(* Logix 5000 AddOnInstructionDefinition export AMCI_MA_Run_Dwell_Move; software revision 20.05 *)

TYPE AMCI_Motion_Axis_Output_Data :
STRUCT
   Control_Word_0 : INT;
   Control_Word_1 : INT;
   Position_or_Distance : DINT;
   Programmed_Speed : DINT;
   Acceleration : INT;
   Deceleration : INT;
   Output_Word_8 : INT;
   Output_Word_9 : INT;
END_STRUCT
END_TYPE

TYPE AMCI_Motion_Axis_Input_Data :
STRUCT
   Moving_CW : BOOL;
   Moving_CCW : BOOL;
   In_Hold_State : BOOL;
   Stopped : BOOL;
   At_Home : BOOL;
   Accelerating : BOOL;
   Decelerating : BOOL;
   Move_Complete : BOOL;
   Status_Word_0_Bit_8 : BOOL;
   Status_Word_0_Bit_9 : BOOL;
   Position_Invalid : BOOL;
   Input_Error : BOOL;
   Command_Error : BOOL;
   Configuration_Error : BOOL;
   Module_OK : BOOL;
   Mode_Flag : BOOL;
   IN1_Active : BOOL;
   IN2_Active : BOOL;
   IN3_Active : BOOL;
   IN4_Active : BOOL;
   Status_Word_1_Bit_4 : BOOL;
   Status_Word_1_Bit_5 : BOOL;
   Connection_Was_Lost : BOOL;
   Driver_Fault : BOOL;
   Status_Word_1_Bit_8 : BOOL;
   Invalid_Jog_Change : BOOL;
   Status_Word_1_Bit_10 : BOOL;
   Heartbeat_Bit : BOOL;
   Status_Word_1_Bit_12 : BOOL;
   Status_Word_1_Bit_13 : BOOL;
   Stall_Detected : BOOL;
   Drive_Is_Enabled : BOOL;
   Motor_Position : DINT;
   Encoder_Position : DINT;
   Trapped_Encoder_Position : DINT;
   Input_Word_8 : INT;
   Input_Word_9 : INT;
END_STRUCT
END_TYPE

ADD_ON_INSTRUCTION AMCI_MA_Run_Dwell_Move   (* revision 1.0, vendor AMCI, ExecuteEnableInFalse *)
// Run Dwell Moves for SD and SMD devices.  Will not work with SV integrated servo devices.
// Help:
// MOTION AXIS RUN DWELL MOVE
// This AOI will only work with the SD and SMD motion devices.  The SV motion devices do not support Assembled Moves.
// AXIS INPUT DATA:  Input data from AMCI motion device.   Uses the AMCI_Motion_Axis_Input_Data User Defined Data Type.
// AXIS OUTPUT DATA; Output data from the AOI to the AMCI motion device.   Uses the AMCI_Motion_Axis_Output_Data User Defined Data Type.
// DWELL TIME:Time in milliseconds between each of the assembled move segments.
// EN (Enable) Set when rung is true, Reset when rung is false
// DN (Done) Set when command is sent to the motion device.  Reset when the rung is false.
// ER (Error) Set when a command or input error failed to clear.  Reset when the rung is false.
// IP (In Process) Set when motion is occurring.   Reset when motion stops or the rung goes false.
VAR_IN_OUT
   Axis_Input_Data : AMCI_Motion_Axis_Input_Data; {required}
   Axis_Output_Data : AMCI_Motion_Axis_Output_Data; {required}
END_VAR
VAR_INPUT
   Type_0_for_standard_1_for_indexed : BOOL;
   Dwell_Time : INT; {required}
END_VAR
VAR_OUTPUT
   EN : BOOL; {visible}
   DN : BOOL; {visible}
   ER : BOOL; {visible}
   IP : BOOL; {visible}
END_VAR
VAR
   command_data_block : INT[10];
        [0]   // Command Bits MSW
        [1]   // Command Bits LSW
        [2]   // Upper Target Position
        [3]   // Lower Target Position
        [4]   // Upper Programmed Speed
        [5]   // Lower Programmed Speed
END_VAR

ROUTINE EnableInFalse   (* ladder *)
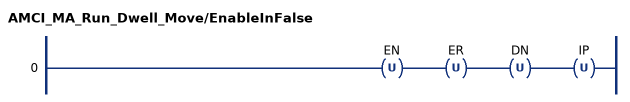
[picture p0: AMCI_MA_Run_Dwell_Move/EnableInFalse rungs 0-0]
   0: OTU(EN)OTU(ER)OTU(DN)OTU(IP);
END_ROUTINE

ROUTINE Logic   (* ladder *)
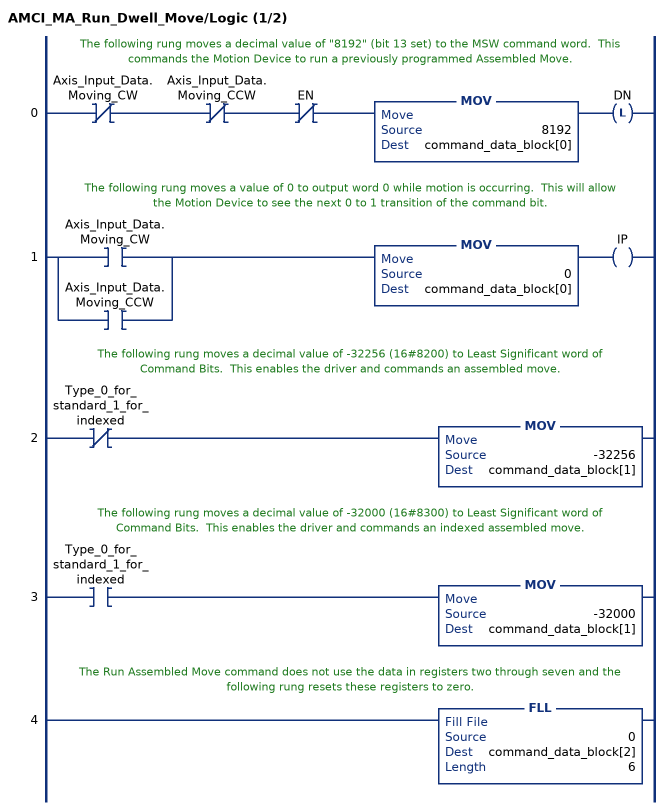
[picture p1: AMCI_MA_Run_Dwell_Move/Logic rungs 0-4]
   // The following rung moves a decimal value of "8192" (bit 13 set) to the MSW command word.  This commands the Motion Device to run a previously programmed Assembled Move.
   0: XIO(Axis_Input_Data.Moving_CW)XIO(Axis_Input_Data.Moving_CCW)XIO(EN)MOV(8192,command_data_block[0])OTL(DN);
   // The following rung moves a value of 0 to output word 0 while motion is occurring.  This will allow the Motion Device to see the next 0 to 1 transition of the command bit.
   1: [XIC(Axis_Input_Data.Moving_CW) ,XIC(Axis_Input_Data.Moving_CCW) ]MOV(0,command_data_block[0])OTE(IP);
   // The following rung moves a decimal value of -32256 (16#8200) to Least Significant word of Command Bits.  This enables the driver and commands an assembled move.
   2: XIO(Type_0_for_standard_1_for_indexed)MOV(-32256,command_data_block[1]);
   // The following rung moves a decimal value of -32000 (16#8300) to Least Significant word of Command Bits.  This enables the driver and commands an indexed assembled move.
   3: XIC(Type_0_for_standard_1_for_indexed)MOV(-32000,command_data_block[1]);
   // The Run Assembled Move command does not use the data in registers two through seven and the following rung resets these registers to zero.
   4: FLL(0,command_data_block[2],6);
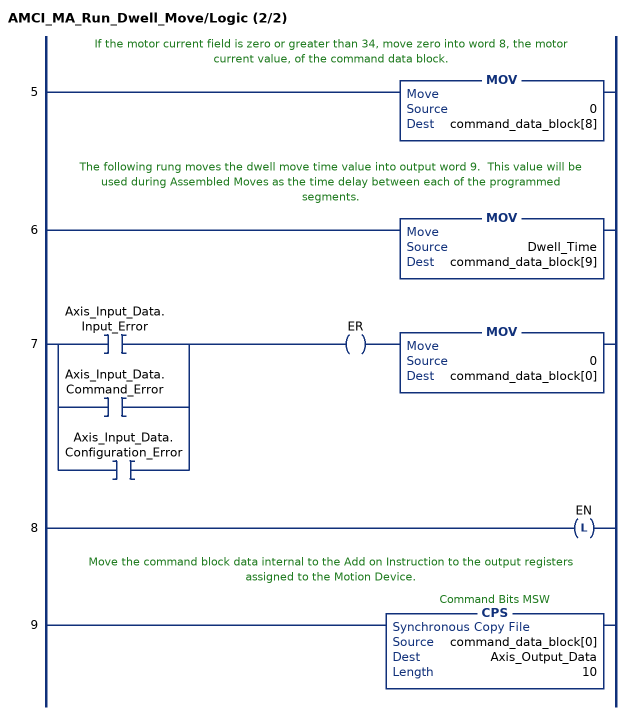
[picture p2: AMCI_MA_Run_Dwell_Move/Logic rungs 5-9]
   // If the motor current field is zero or greater than 34, move zero into word 8, the motor current value, of the command data block.
   5: MOV(0,command_data_block[8]);
   // The following rung moves the dwell move time value into output word 9.  This value will be used during Assembled Moves as the time delay between each of the programmed segments.
   6: MOV(Dwell_Time,command_data_block[9]);
   7: [XIC(Axis_Input_Data.Input_Error) ,XIC(Axis_Input_Data.Command_Error) ,XIC(Axis_Input_Data.Configuration_Error) ]OTE(ER)MOV(0,command_data_block[0]);
   8: OTL(EN);
   // Move the command block data internal to the Add on Instruction to the output registers assigned to the Motion Device.
   9: CPS(command_data_block[0],Axis_Output_Data,10);
END_ROUTINE
END_ADD_ON_INSTRUCTION
